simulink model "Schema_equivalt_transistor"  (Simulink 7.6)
settings: Solver=ode15s  StartTime=0.0  StopTime=5e-3  RelTol=1e-3
InitFcn:
  | h11=1e3;
  | h12=5e-4;
  | h21=100;
  | h22=5e-5;
  | 
  | Rc=10e3;
  | Rb=47e3;
StopFcn:
  | close all
  | load es.mat
  | plot(es(1,:),es(2,:),'r',es(1,:),es(3,:))
  | title('Schéma équivalent du transistor')
  | 
  | axis([0 5e-3 -12 12])
  | grid
libraries: fl_lib x16, nesl_utility x3

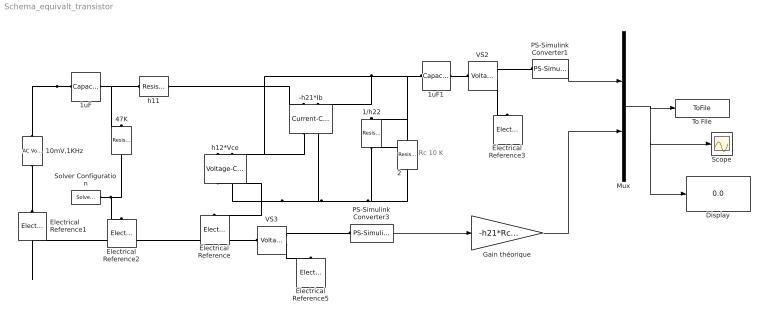
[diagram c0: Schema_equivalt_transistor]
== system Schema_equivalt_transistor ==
  note: Rc 10 K
  -h21*Ib : fl_lib/Electrical/Electrical Sources/Current-Controlled Current Source  DialogController=NetworkEngine.DynNeDlgSource  SystemSampleTime=-1  K=-h21  i1_Log=off  v1_Log=off  i2_Log=off  v2_Log=off  LocalVarNames=|input_current|output_voltage|output_current|output_power  LocalVarDescs=|Input current (A)|Output voltage (V)|Output current (A)|Output power (W)  LocalVarLogging=[0 0 0 0]
  1/h22 : fl_lib/Electrical/Electrical Elements/Resistor  DialogController=NetworkEngine.DynNeDlgSource  SystemSampleTime=-1  R=1/h22 Ohm  i_Log=off  v_Log=off  LocalVarNames=|current|voltage|power  LocalVarDescs=|Resistor current (A)|Voltage across resistor (V)|Power (W)  LocalVarLogging=[0 0 0]
  10mV,1KHz : fl_lib/Electrical/Electrical Sources/AC Voltage Source  DialogController=NetworkEngine.DynNeDlgSource  SystemSampleTime=-1  amp=0.01 V  shift=0 rad  omega=1000 Hz  i_Log=off  v_Log=off  LocalVarNames=|current|voltage|power  LocalVarDescs=|Current (A)|Voltage (V)|Power (W)  LocalVarLogging=[0 0 0]
  1uF : fl_lib/Electrical/Electrical Elements/Capacitor  DialogController=NetworkEngine.DynNeDlgSource  SystemSampleTime=-1  c=1e-06 F  v0=0 V  r=1e-06 Ohm  g=0 1/Ohm  i_Log=off  v_Log=off  vc_Log=off  LocalVarNames=|current|voltage|power  LocalVarDescs=|Capacitor current (A)|Voltage across capacitor (V)|Power (W)  LocalVarLogging=[0 0 0]
  1uF1 : fl_lib/Electrical/Electrical Elements/Capacitor  DialogController=NetworkEngine.DynNeDlgSource  SystemSampleTime=-1  c=100e-06 F  v0=0 V  r=1e-06 Ohm  g=0 1/Ohm  i_Log=off  v_Log=off  vc_Log=off  LocalVarNames=|current|voltage|power  LocalVarDescs=|Capacitor current (A)|Voltage across capacitor (V)|Power (W)  LocalVarLogging=[0 0 0]
  2 : fl_lib/Electrical/Electrical Elements/Resistor  DialogController=NetworkEngine.DynNeDlgSource  SystemSampleTime=-1  R=Rc Ohm  i_Log=off  v_Log=off  LocalVarNames=|current|voltage|power  LocalVarDescs=|Resistor current (A)|Voltage across resistor (V)|Power (W)  LocalVarLogging=[0 0 0]
  47K : fl_lib/Electrical/Electrical Elements/Resistor  DialogController=NetworkEngine.DynNeDlgSource  SystemSampleTime=-1  R=Rb Ohm  i_Log=off  v_Log=off  LocalVarNames=|current|voltage|power  LocalVarDescs=|Resistor current (A)|Voltage across resistor (V)|Power (W)  LocalVarLogging=[0 0 0]
  Display : Display
  Electrical Reference{,1..3,5} (5 alike) : fl_lib/Electrical/Electrical Elements/Electrical Reference  DialogController=NetworkEngine.DynNeDlgSource  SystemSampleTime=-1  i_Log=off  LocalVarNames=|i  LocalVarDescs=|i  LocalVarLogging=[]
  Gain théorique : Gain  Gain=-h21*Rc/h11
  Mux : Mux  Inputs=2
  PS-Simulink Converter1 : nesl_utility/PS-Simulink Converter  DialogController=NetworkEngine.DynNeUtilDlgSource  SystemSampleTime=-1  PhysicalDomain=network_engine_domain  LeftPortType=input  RightPortType=output  SubClassName=ps_output  Unit=1  AffineConversion=off
  PS-Simulink Converter3 : nesl_utility/PS-Simulink Converter  DialogController=NetworkEngine.DynNeUtilDlgSource  SystemSampleTime=-1  PhysicalDomain=network_engine_domain  LeftPortType=input  RightPortType=output  SubClassName=ps_output  Unit=1  AffineConversion=off
  Scope : Scope
  Solver Configuration : nesl_utility/Solver Configuration  DialogController=NetworkEngine.DynNeUtilDlgSource  SystemSampleTime=-1  PhysicalDomain=network_engine_domain  LeftPortType=input  RightPortType=generic  SubClassName=solver  Accelerate=off  Profile=off  ResidualTolerance=1e-9  MaxNonlinIter=12  MaxModeIter=2  DoFixedCost=off  UseLocalSampling=off  DoDC=off  LinearAlgebra=Sparse  LocalSolverSampleTime=.001  LocalSolverChoice=NE_BACKWARD_EULER_ADVANCER  UseLocalSolver=off
  To File : ToFile  Filename=es.mat  MatrixName=es
  VS2 : fl_lib/Electrical/Electrical Sensors/Voltage Sensor  DialogController=NetworkEngine.DynNeDlgSource  SystemSampleTime=-1  i1_Log=off  v1_Log=off  LocalVarNames=|i1|v1  LocalVarDescs=|i1|v1  LocalVarLogging=[]
  VS3 : fl_lib/Electrical/Electrical Sensors/Voltage Sensor  DialogController=NetworkEngine.DynNeDlgSource  SystemSampleTime=-1  i1_Log=off  v1_Log=off  LocalVarNames=|i1|v1  LocalVarDescs=|i1|v1  LocalVarLogging=[]
  h11 : fl_lib/Electrical/Electrical Elements/Resistor  DialogController=NetworkEngine.DynNeDlgSource  SystemSampleTime=-1  R=h11 Ohm  i_Log=off  v_Log=off  LocalVarNames=|current|voltage|power  LocalVarDescs=|Resistor current (A)|Voltage across resistor (V)|Power (W)  LocalVarLogging=[0 0 0]
  h12*Vce : fl_lib/Electrical/Electrical Sources/Voltage-Controlled Voltage Source  DialogController=NetworkEngine.DynNeDlgSource  SystemSampleTime=-1  K=h12  i1_Log=off  v1_Log=off  i2_Log=off  v2_Log=off  LocalVarNames=|input_voltage|output_voltage|output_current|output_power  LocalVarDescs=|Input voltage (V)|Output voltage (V)|Output current (A)|Output power (W)  LocalVarLogging=[0 0 0 0]
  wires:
  Mux/1 -> To File/1, Scope/1, Display/1
  PS-Simulink Converter3/1 -> Gain théorique/1
  PS-Simulink Converter1/1 -> Mux/1
  Gain théorique/1 -> Mux/2
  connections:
  h12*Vce/LConn1 -- -h21*Ib/LConn2 -- 1/h22/LConn1 -- 2/RConn1 -- 1uF1/LConn1
  h12*Vce/RConn1 -- Electrical Reference/LConn1 -- h12*Vce/RConn2 -- -h21*Ib/RConn2 -- 1/h22/RConn1 -- 2/LConn1
  1uF/RConn1 -- h11/LConn1 -- 47K/LConn1
  -h21*Ib/RConn1 -- h12*Vce/LConn2
  h11/RConn1 -- -h21*Ib/LConn1
  10mV,1KHz/RConn1 -- Electrical Reference1/LConn1
  1uF1/RConn1 -- VS2/LConn1
  VS2/RConn2 -- Electrical Reference3/LConn1
  VS2/RConn1 -- PS-Simulink Converter1/LConn1
  Solver Configuration/RConn1 -- Electrical Reference2/LConn1 -- 47K/RConn1
  VS3/RConn2 -- Electrical Reference5/LConn1
  VS3/RConn1 -- PS-Simulink Converter3/LConn1
  10mV,1KHz/LConn1 -- 1uF/LConn1 -- VS3/LConn1
